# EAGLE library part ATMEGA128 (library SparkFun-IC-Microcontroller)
ATmega 128 ATmega128/128L/1281/2561. Note: The ATmega128 pin 1 is PEN and the ATmega256/1281 pin 1 is PG5. Not in catalog
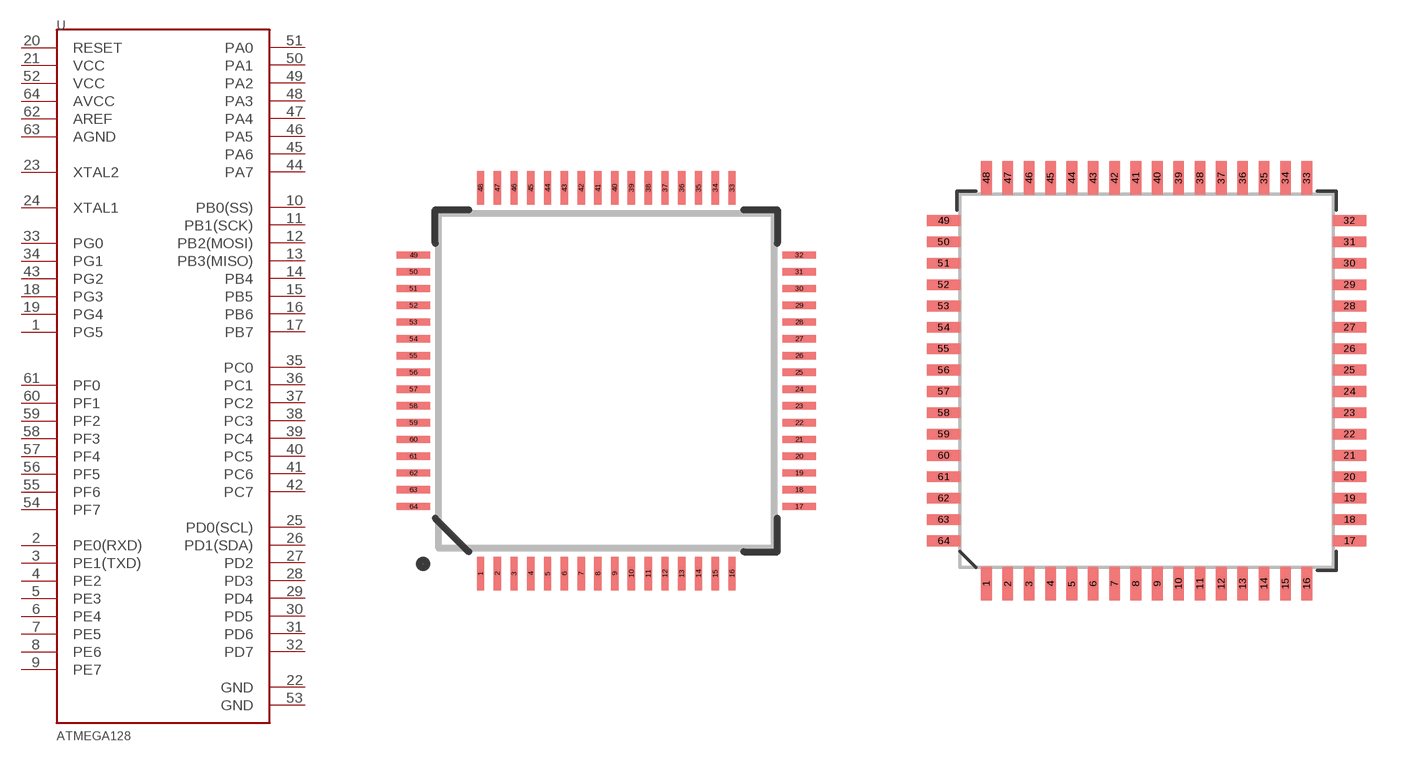
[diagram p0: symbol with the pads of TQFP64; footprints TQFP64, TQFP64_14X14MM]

Designator prefix U

## ATMEGA128_SMD  [TQFP64]
1  PG5
2  PE0(RXD)
3  PE1(TXD)
4  PE2
5  PE3
6  PE4
7  PE5
8  PE6
9  PE7
10  PB0(SS)
11  PB1(SCK)
12  PB2(MOSI)
13  PB3(MISO)
14  PB4
15  PB5
16  PB6
17  PB7
18  PG3
19  PG4
20  RESET
21  VCC
22  GND
23  XTAL2
24  XTAL1
25  PD0(SCL)
26  PD1(SDA)
27  PD2
28  PD3
29  PD4
30  PD5
31  PD6
32  PD7
33  PG0
34  PG1
35  PC0
36  PC1
37  PC2
38  PC3
39  PC4
40  PC5
41  PC6
42  PC7
43  PG2
44  PA7
45  PA6
46  PA5
47  PA4
48  PA3
49  PA2
50  PA1
51  PA0
52  VCC
53  GND
54  PF7
55  PF6
56  PF5
57  PF4
58  PF3
59  PF2
60  PF1
61  PF0
62  AREF
63  AGND
64  AVCC

## ATMEGA128-SMD  [TQFP64_14X14MM]
Pads as for TQFP64

## Footprint TQFP64 (pad centres in mm)
64-Lead TQFP Plastic Thin Quad Flatpack - 10x10x1mm Body, 2mmFP
smd 0.22 x 1: 1 -3.75,-5.75; 2 -3.25,-5.75; 3 -2.75,-5.75; 4 -2.25,-5.75; 5 -1.75,-5.75; 6 -1.25,-5.75; 7 -0.75,-5.75; 8 -0.25,-5.75; 9 0.25,-5.75; 10 0.75,-5.75; 11 1.25,-5.75; 12 1.75,-5.75; 13 2.25,-5.75; 14 2.75,-5.75; 15 3.25,-5.75; 16 3.75,-5.75; 33 3.75,5.75; 34 3.25,5.75; 35 2.75,5.75; 36 2.25,5.75; 37 1.75,5.75; 38 1.25,5.75; 39 0.75,5.75; 40 0.25,5.75; 41 -0.25,5.75; 42 -0.75,5.75; 43 -1.25,5.75; 44 -1.75,5.75; 45 -2.25,5.75; 46 -2.75,5.75; 47 -3.25,5.75; 48 -3.75,5.75
smd 1 x 0.22: 17 5.75,-3.75; 18 5.75,-3.25; 19 5.75,-2.75; 20 5.75,-2.25; 21 5.75,-1.75; 22 5.75,-1.25; 23 5.75,-0.75; 24 5.75,-0.25; 25 5.75,0.25; 26 5.75,0.75; 27 5.75,1.25; 28 5.75,1.75; 29 5.75,2.25; 30 5.75,2.75; 31 5.75,3.25; 32 5.75,3.75; 49 -5.75,3.75; 50 -5.75,3.25; 51 -5.75,2.75; 52 -5.75,2.25; 53 -5.75,1.75; 54 -5.75,1.25; 55 -5.75,0.75; 56 -5.75,0.25; 57 -5.75,-0.25; 58 -5.75,-0.75; 59 -5.75,-1.25; 60 -5.75,-1.75; 61 -5.75,-2.25; 62 -5.75,-2.75; 63 -5.75,-3.25; 64 -5.75,-3.75

## Footprint TQFP64_14X14MM (pad centres in mm)
64-Lead TQFP Plastic Thin Quad Flatpack - 14x14x1mm Body
smd 0.4 x 1.27: 1 -6,-7.6; 2 -5.2,-7.6; 3 -4.4,-7.6; 4 -3.6,-7.6; 5 -2.8,-7.6; 6 -2,-7.6; 7 -1.2,-7.6; 8 -0.4,-7.6; 9 0.4,-7.6; 10 1.2,-7.6; 11 2,-7.6; 12 2.8,-7.6; 13 3.6,-7.6; 14 4.4,-7.6; 15 5.2,-7.6; 16 6,-7.6; 33 6,7.6; 34 5.2,7.6; 35 4.4,7.6; 36 3.6,7.6; 37 2.8,7.6; 38 2,7.6; 39 1.2,7.6; 40 0.4,7.6; 41 -0.4,7.6; 42 -1.2,7.6; 43 -2,7.6; 44 -2.8,7.6; 45 -3.6,7.6; 46 -4.4,7.6; 47 -5.2,7.6; 48 -6,7.6
smd 1.27 x 0.4: 17 7.6,-6; 18 7.6,-5.2; 19 7.6,-4.4; 20 7.6,-3.6; 21 7.6,-2.8; 22 7.6,-2; 23 7.6,-1.2; 24 7.6,-0.4; 25 7.6,0.4; 26 7.6,1.2; 27 7.6,2; 28 7.6,2.8; 29 7.6,3.6; 30 7.6,4.4; 31 7.6,5.2; 32 7.6,6; 49 -7.6,6; 50 -7.6,5.2; 51 -7.6,4.4; 52 -7.6,3.6; 53 -7.6,2.8; 54 -7.6,2; 55 -7.6,1.2; 56 -7.6,0.4; 57 -7.6,-0.4; 58 -7.6,-1.2; 59 -7.6,-2; 60 -7.6,-2.8; 61 -7.6,-3.6; 62 -7.6,-4.4; 63 -7.6,-5.2; 64 -7.6,-6

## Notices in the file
Licensing: Creative Commons ShareAlike 4.0 International - https://creativecommons.org/licenses/by-sa/4.0
